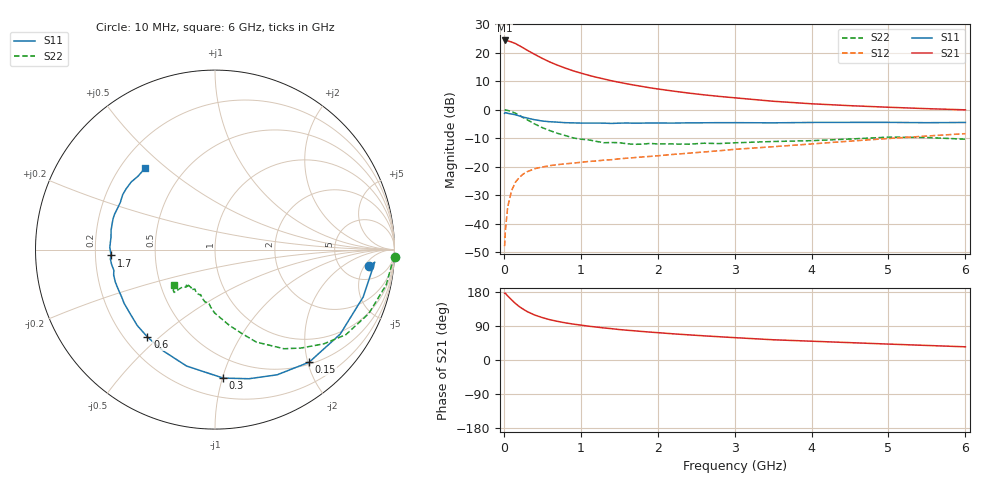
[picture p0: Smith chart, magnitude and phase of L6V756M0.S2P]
!  INFINEON TECHNOLOGIES Small Signal Semiconductors
! BFR380L3 , Si-NPN RF-Transistor in TSLP-3-1
!  Vce=0.75 V,  Ic=6 mA
! Common Emitter S-Parameters:  07. March 2005
#  GHz  S  MA  R  50
! f  S11  S21  S12  S22
! GHz  Mag  Ang  Mag  Ang  Mag  Ang  Mag  Ang
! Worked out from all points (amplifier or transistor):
!   36 points, 10 MHz to 6 GHz, reference 50 ohm
!   highest |S21| = 24.4 dB at 10 MHz (marker M1)
!   |S21| within 3 dB of that: start of sweep to 276.6 MHz
!   unconditionally stable (mu >= 1): 2.204 GHz to 4.997 GHz
!   at 250 MHz: K = 0.20, MSG = 22.2 dB, |S12| = -22.6 dB
!   at 1.4 GHz: K = 0.83, MSG = 13.9 dB, |S12| = -17.5 dB
!   at 6 GHz: K = 0.98, MSG = 4.2 dB, |S12| = -8.4 dB
!   S11 on the Smith chart (normalised r, x): 10 MHz: 9, -6; 150 MHz: 0.53, -2.03; 300 MHz: 0.34, -1.01; 600 MHz: 0.29, -0.46; 1.7 GHz: 0.27, -0.03; 6 GHz: 0.30, +0.43
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0.01  0.8649 -5.9  16.53 176.1  0.004 82.3  1.006 -2.4
0.02  0.8926 -4.5  16.4 176.0  0.0075 85.6  0.9886 -4.8
0.05  0.8669 -17.7  16.28 169.0  0.0195 81.4  0.974 -11.6
0.1  0.8417 -34.0  15.53 158.9  0.0377 73.5  0.9279 -22.6
0.15  0.8178 -50.1  14.59 149.3  0.0531 65.4  0.8698 -33.0
0.2  0.7788 -63.6  13.42 141.0  0.0643 59.3  0.8019 -40.9
0.25  0.7438 -75.3  12.3 134.3  0.0738 54.4  0.7288 -48.8
0.3  0.7172 -86.4  11.21 128.1  0.0811 50.4  0.6727 -55.2
0.4  0.6675 -103.8  9.422 118.7  0.092 44.8  0.5636 -66.0
0.5  0.6341 -116.9  8.008 111.9  0.0986 41.8  0.4853 -72.8
0.6  0.6154 -127.7  6.891 106.2  0.1043 40.1  0.4293 -79.3
0.7  0.6054 -135.7  6.06 101.9  0.1084 39.5  0.3847 -85.0
0.8  0.5925 -142.9  5.397 98.0  0.1122 39.1  0.3518 -90.5
1.1  0.5828 -157.8  4.046 89.3  0.1232 40.3  0.2958 -101.0
1.4  0.5751 -168.4  3.236 82.7  0.1326 42.2  0.2657 -108.6
1.7  0.5805 -176.8  2.703 77.0  0.1444 44.6  0.247 -116.7
2.2  0.5834 173.1  2.131 69.1  0.1641 48.2  0.2503 -121.7
2.8  0.5934 163.1  1.718 61.4  0.1904 52.0  0.2546 -128.8
3.5  0.5892 153.6  1.412 53.4  0.224 53.8  0.2766 -130.7
4.5  0.5999 145.8  1.18 45.8  0.281 56.2  0.3058 -132.7
5.5  0.5927 136.3  1.046 38.4  0.3454 55.1  0.3253 -135.5
6  0.5984 130.4  0.997 34.8  0.3804 53.8  0.3035 -139.1
